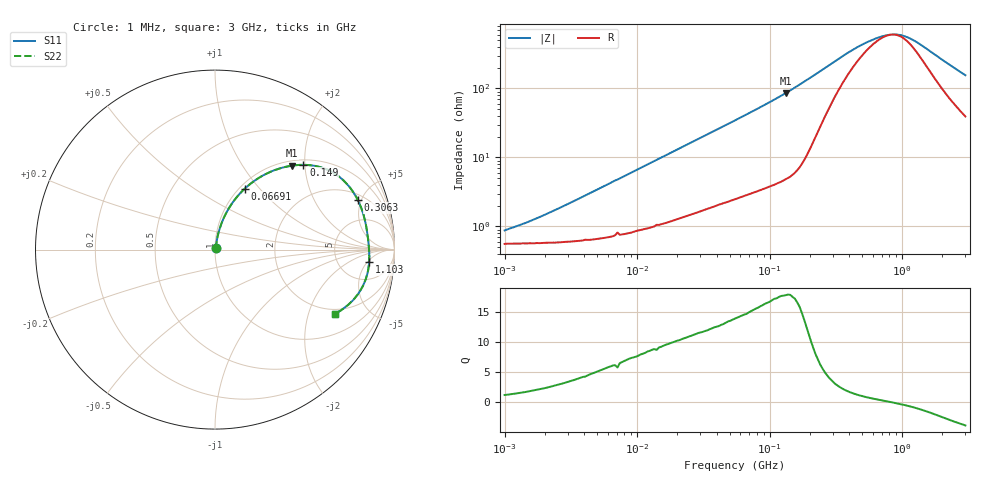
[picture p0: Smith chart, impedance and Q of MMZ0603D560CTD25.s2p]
! S-Parameter Data Generated by TDK Corporation
! Copyright(C) 2025 TDK Corporation.
! All Rights Reserved.
! TDK P/N: MMZ0603D560CTD25 (Chip Bead)
! Property: |Z|=56ohm at 100MHz
! Size(LxWxT): 0.6x0.3x0.3mm
! Model Type: s2p (Touchstone File Format Version 1.0)
! Frequency: DC=Yes Start=1MHz Stop=3000MHz 202points Log-sweep
! Model Generated on Feb. 6, 2025
! Terms and conditions regarding TDK Simulation Models:
! 1)This simulation model is being provided solely for informational
!  purposes. Please refer to the specifications of the products in
!  terms of detailed characteristics of such products.
! 2)In no event shall TDK Corporation of any of its subsidiaries be
!  liable for any loss or damage arising, directly or indirectly,
!  from any information contained in this simulation model, including,
!  but not limited to loss or damages arising from any inaccuracies,
!  omissions or errors in connection with such information.
! 3)Any and all copyrights on this simulation model are owned by
!  TDK Corporation.  Duplication or redistribution of this simulation
!  model without prior written permission from TDK Corporation
!  is prohibited.
! 4)This simulation model is subject to any modification or change
!  without any prior notice.
! 5)Neither TDK Corporation nor any of its subsidiaries shall make any
!  warranty, express or implied, including but not limited to the
!  correctness, implied warranties of merchantability and fitness for
!  a particular purpose with respect to this simulation models.
! 6)The use of this simulation model shall be deemed to have consented
!  to the terms and conditions hereof.
! Port Assignments:
!  1 ---@@@--- 2
! Applicable Conditions:
!  Temperature = 25 degC
!  DC Bias Current = 0 A
!  Small Signal Operation
# Hz S MA R 50
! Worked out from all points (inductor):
!   201 points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, 1 MHz to 3 GHz, reference 50 ohm
!   read as one part in series: L = 107 nH near 2.614 MHz
!   highest Q = 17.8 at 132.1 MHz (marker M1), where L = 103 nH
!   self-resonance near 836.6 MHz
!   S11 on the Smith chart (normalised r, x): 1 MHz: 1.01, +0.01; 66.91 MHz: 1.06, +0.84; 149 MHz: 1.11, +1.97; 306.3 MHz: 2.44, +4.66; 1.103 GHz: 11, -6; 3 GHz: 1.79, -3.01
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1000000  0.008703 50.1  0.9944 -0.4  0.9944 -0.4  0.008703 50.1
1822989  0.01348 64.4  0.9942 -0.7  0.9942 -0.7  0.01348 64.4
3900413  0.02685 75.1  0.9935 -1.5  0.9935 -1.5  0.02685 75.1
1.461624e7  0.0945 78.3  0.9852 -5.4  0.9852 -5.4  0.0945 78.3
3.127247e7  0.1926 74.0  0.965 -11.1  0.965 -11.1  0.1926 74.0
5.477226e7  0.3187 67.3  0.9252 -18.5  0.9252 -18.5  0.3187 67.3
6.690963e7  0.3781 63.9  0.9004 -22.2  0.9004 -22.2  0.3781 63.9
9.593103e7  0.5048 56.3  0.8332 -30.3  0.8332 -30.3  0.5048 56.3
1.321429e8  0.6333 47.6  0.7391 -39.2  0.7391 -39.2  0.6333 47.6
1.49005e8  0.6822 43.8  0.6932 -42.9  0.6932 -42.9  0.6822 43.8
1.748812e8  0.7424 38.4  0.622 -47.8  0.622 -47.8  0.7424 38.4
2.136344e8  0.7978 31.2  0.5211 -52.5  0.5211 -52.5  0.7978 31.2
3.062963e8  0.8418 19.3  0.3453 -53.5  0.3453 -53.5  0.8418 19.3
5.364635e8  0.8533 6.9  0.1837 -33.7  0.1837 -33.7  0.8533 6.9
6.553423e8  0.8549 3.7  0.1568 -20.5  0.1568 -20.5  0.8549 3.7
8.005644e8  0.8576 0.7  0.1428 -4.0  0.1428 -4.0  0.8576 0.7
9.779672e8  0.8608 -2.5  0.1448 14.8  0.1448 14.8  0.8608 -2.5
1.10276e9  0.8616 -4.5  0.1565 25.7  0.1565 25.7  0.8616 -4.5
1.294266e9  0.8611 -7.5  0.1841 37.4  0.1841 37.4  0.8611 -7.5
1.855641e9  0.8427 -15.3  0.2909 49.9  0.2909 49.9  0.8427 -15.3
2.359433e9  0.8107 -21.4  0.3844 50.4  0.3844 50.4  0.8107 -21.4
3e9  0.759 -28.1  0.4873 47.3  0.4873 47.3  0.759 -28.1
